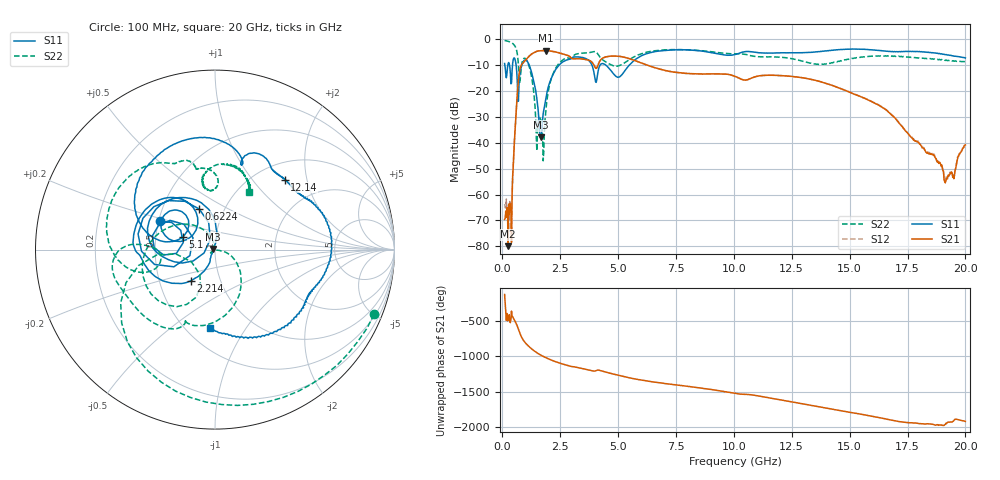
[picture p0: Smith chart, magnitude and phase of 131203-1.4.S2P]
!  2-Port S-parameters saved by WinCal
! VAR MeasName=S-Parameters (CALIBRATED_DATA) read from VNA (N5244A)
! VAR MeasDate=4/4/2013 3:55:45 PM
! VAR NAME=131203-1.4
! VAR FILENAME=131203-1.4.S2P
! VAR DATE=4/4/2013 3:55:45 PM
! VAR PHYS_PORTS=1,2
# Hz S MA R 50
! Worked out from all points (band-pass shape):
!   801 points, 100 MHz to 20 GHz, reference 50 ohm
!   highest |S21| = -4.27 dB at 1.891 GHz (marker M1); lowest = -80.0 dB at 249.2 MHz (marker M2)
!   |S21| within 3 dB of the highest: 1.078 GHz to 2.992 GHz (1.915 GHz wide, 94.1 % of centre); 4.328 GHz to 5.435 GHz (1.107 GHz wide, 22.7 % of centre)
!   lowest |S11| = -37.8 dB at 1.667 GHz (marker M3), VSWR 1.03, Z = 48.8 + j0.338 ohm
!   |S11| at or under -10 dB: 1.166 GHz to 2.446 GHz (1.279 GHz wide, 70.8 % of centre); 3.874 GHz to 4.217 GHz (343.4 MHz wide, 8.49 % of centre); 4.481 GHz to 5.476 GHz (995.6 MHz wide, 20 % of centre)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
!   |S22| runs from -47.0 to -0.4 dB; largest |S21 - S12| = 0.0025
!   S11 on the Smith chart (normalised r, x): 100 MHz: 0.51, +0.18; 622.4 MHz: 0.76, +0.37; 2.214 GHz: 0.72, -0.26; 5.1 GHz: 0.69, +0.10; 12.14 GHz: 1.32, +1.48; 20 GHz: 0.65, -0.70
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1e8  0.3424 152.6  0.0003309 -128.8  0.0006548 -168.4  0.9571 -22.2
2.4925e8  0.3389 178.2  0.0001002 -130.4  0.0004264 -140.2  0.9224 -54.2
3.73625e8  0.1386 151.9  0.0005419 -114.8  0.0002273 -128.7  0.8772 -81.8
6.22375e8  0.2429 111.2  0.05872 165.4  0.05865 166.0  0.6036 -150.5
8.71125e8  0.3473 178.4  0.3443 -34.4  0.3451 -34.3  0.3824 -123.7
1.14475e9  0.3338 119.8  0.4669 -141.7  0.4678 -141.7  0.3172 161.6
1.468125e9  0.08535 82.6  0.584 134.3  0.5855 134.3  0.0131 103.1
1.667125e9  0.01283 164.3  0.6045 94.3  0.6063 94.2  0.02751 -143.6
1.7915e9  0.04281 -122.0  0.6089 72.8  0.6106 72.8  0.006802 -31.9
1.891e9  0.07793 -112.2  0.6115 57.1  0.6131 57.1  0.04671 -12.4
2.214375e9  0.2209 -127.9  0.5842 12.5  0.5859 12.4  0.2297 -50.5
2.761625e9  0.3974 -166.8  0.5012 -45.9  0.5024 -45.9  0.4349 -103.1
3.43325e9  0.4505 152.9  0.4201 -93.4  0.4207 -93.3  0.5423 -138.2
4.204375e9  0.3088 161.1  0.376 -120.1  0.3777 -120.3  0.4637 176.4
5.099875e9  0.1945 158.4  0.4687 163.0  0.47 163.0  0.3173 -166.1
6.741625e9  0.5957 130.9  0.2718 65.6  0.272 65.4  0.6156 168.8
1.005e10  0.5124 73.4  0.1937 -86.8  0.1933 -86.8  0.5297 113.3
1.21395e10  0.5507 45.2  0.1989 175.0  0.1983 175.4  0.448 94.3
1.338325e10  0.5644 33.0  0.1675 101.0  0.1676 101.3  0.3409 89.2
1.669162e10  0.5849 -22.6  0.03872 -96.7  0.03966 -96.2  0.4741 78.5
1.917912e10  0.5099 -74.3  0.002036 -153.9  0.002251 -146.7  0.3995 61.2
2e10  0.4388 -93.8  0.009107 -122.4  0.009413 -123.8  0.3728 59.2
